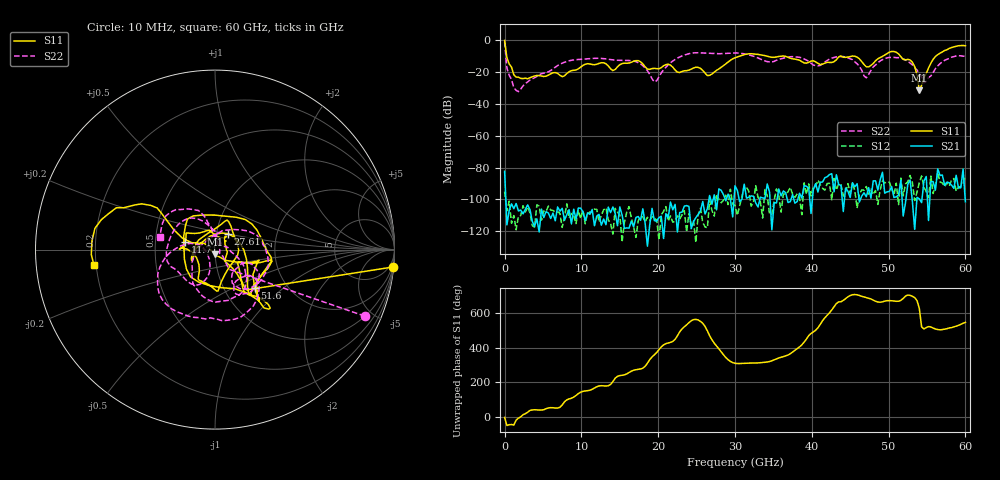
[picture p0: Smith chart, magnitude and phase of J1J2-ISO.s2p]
!Keysight Technologies,N5227A,US51270214,A.10.65.11
!Date: Thursday, October 15, 2020 08:21:50
!Correction: S11(Full 2 Port(1,2))
!S21(Full 2 Port(1,2))
!S12(Full 2 Port(1,2))
!S22(Full 2 Port(1,2))
!S2P File: Measurements: S11, S21, S12, S22:
# Hz S  dB  R 50
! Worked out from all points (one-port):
!   201 points, 10 MHz to 60 GHz, reference 50 ohm
!   lowest |S11| = -31.5 dB at 54 GHz (marker M1), VSWR 1.05, Z = 49.9 - j2.66 ohm
!   |S11| at or under -10 dB: 284.8 MHz to 30.57 GHz (30.29 GHz wide, 196 % of centre); 36.55 GHz to 43.7 GHz (7.149 GHz wide, 17.8 % of centre); 51.56 GHz to 56.13 GHz (4.569 GHz wide, 8.49 % of centre)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
!   S11 on the Smith chart (normalised r, x): 10 MHz: 1, -21; 11.71 GHz: 0.71, +0.06; 27.61 GHz: 1.14, +0.20; 51.6 GHz: 1.39, -0.66; 60 GHz: 0.19, -0.06
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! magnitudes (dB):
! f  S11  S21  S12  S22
! 10 MHz  0.0  -82.4  -95.2  -0.8
! 309.9 MHz  -10.9  -116.1  -107.2  -17.4
! 1.81 GHz  -23.1  -107.3  -110.8  -32.2
! 10.21 GHz  -15.8  -107.9  -106.7  -11.8
! 11.71 GHz  -15.3  -116.7  -106.2  -11.3
! 14.11 GHz  -19.0  -104.9  -121.9  -12.3
! 17.11 GHz  -12.7  -111.4  -124.0  -13.4
! 19.51 GHz  -17.6  -113.4  -112.0  -26.1
! 20.11 GHz  -17.8  -111.5  -125.6  -23.0
! 23.11 GHz  -19.6  -108.1  -109.9  -9.8
! 27.61 GHz  -18.8  -106.7  -96.7  -8.3
! 30 GHz  -10.9  -91.5  -103.8  -7.9
! 40.2 GHz  -12.8  -93.8  -92.0  -15.5
! 44.1 GHz  -10.6  -107.7  -98.0  -10.2
! 47.1 GHz  -16.6  -98.4  -92.0  -23.5
! 50.1 GHz  -7.4  -95.1  -89.2  -10.7
! 51.6 GHz  -10.2  -87.9  -86.7  -11.1
! 53.1 GHz  -13.8  -101.4  -89.5  -15.4
! 54 GHz  -31.5  -99.7  -89.5  -20.9
! 54.6 GHz  -23.3  -88.5  -92.2  -26.8
! 56.1 GHz  -10.1  -94.3  -91.4  -17.7
! 60 GHz  -3.4  -101.6  -85.3  -10.1
